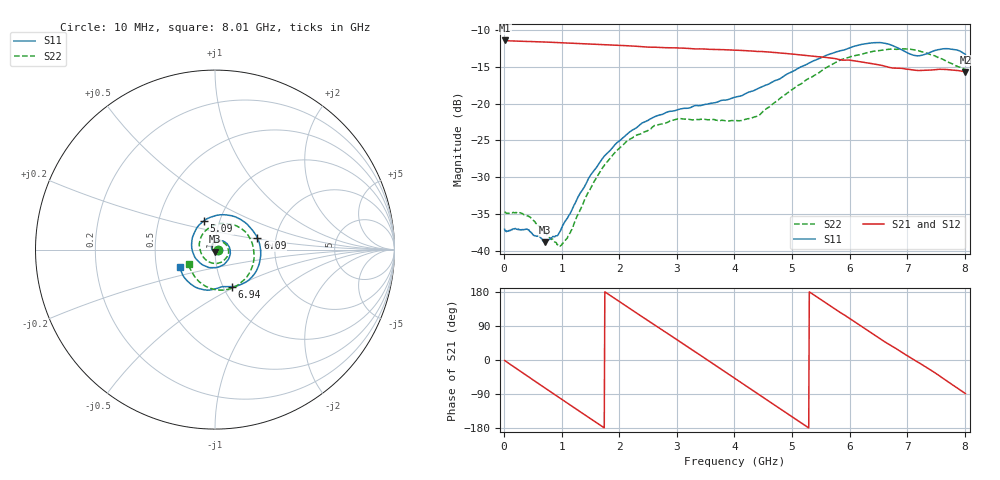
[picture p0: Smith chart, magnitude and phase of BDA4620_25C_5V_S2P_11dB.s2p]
!Agilent Technologies,E5071B,MY42404982,A.09.10
!Date: Wed May 06 09:00:28 2026
!Data & Calibration Information:
!Freq	S11:SOLT2(ON)	S21:SOLT2(ON)	S12:SOLT2(ON)	S22:SOLT2(ON)
# Hz S RI R 50
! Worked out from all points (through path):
!   801 points, 10 MHz to 8.01 GHz, reference 50 ohm
!   highest |S21| = -11.44 dB at 10 MHz (marker M1); lowest = -15.7 dB at 8.01 GHz (marker M2)
!   group delay of S21, straight-line fit = 280 ps
!   lowest |S11| = -38.9 dB at 710 MHz (marker M3), VSWR 1.02, Z = 49.9 - j1.14 ohm
!   |S11| at or under -10 dB: start of sweep to end of sweep
!   |S22| runs from -39.4 to -12.6 dB; largest |S21 - S12| = 0.0012
!   S11 on the Smith chart (normalised r, x): 10 MHz: 1.03, -0.00; 5.09 GHz: 0.84, +0.28; 6.09 GHz: 1.60, +0.22; 6.94 GHz: 1.10, -0.48; 8.01 GHz: 0.67, -0.13
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1e7  0.014 -0.00093  0.2679 -0.0057  0.2683 -0.00581  0.0184 -0.00107
4.2e8  0.00997 -0.00968  0.1902 -0.1827  0.1905 -0.1833  0.0137 -0.0103
7.1e8  -0.000638 -0.0114  0.073 -0.251  0.073 -0.2516  0.0034 -0.013
9.9e8  -0.0131 -0.00478  -0.056 -0.2525  -0.0564 -0.253  -0.0086 -0.00671
1.35e9  -0.0192 0.0169  -0.1938 -0.1659  -0.1939 -0.1661  -0.0153 0.0128
1.67e9  -0.0066 0.0397  -0.249 -0.035  -0.2494 -0.0351  -0.00637 0.034
1.94e9  0.0162 0.0507  -0.2346 0.0825  -0.2349 0.0828  0.0129 0.0455
2.33e9  0.0569 0.0407  -0.1257 0.2093  -0.126 0.2096  0.0475 0.0393
2.68e9  0.0831 0.00493  0.017 0.24  0.0173 0.2403  0.0703 0.0138
3.39e9  0.0393 -0.0885  0.2275 0.0585  0.2279 0.0583  0.046 -0.0628
4.01e9  -0.0738 -0.082  0.1521 -0.1728  0.1523 -0.1732  -0.0452 -0.0619
4.52e9  -0.1306 0.0203  -0.0419 -0.2209  -0.042 -0.2213  -0.0874 0.021
5.09e9  -0.0617 0.1606  -0.2006 -0.0772  -0.2012 -0.0771  -0.0185 0.1303
5.35e9  0.0163 0.1924  -0.2089 0.0192  -0.2091 0.0194  0.0468 0.1443
5.68e9  0.1305 0.1749  -0.1589 0.1271  -0.1588 0.1276  0.1337 0.1246
6.09e9  0.2367 0.0646  -0.0341 0.1918  -0.0343 0.1923  0.2099 0.0263
6.39e9  0.2505 -0.062  0.0641 0.1751  0.0641 0.1753  0.2157 -0.0652
6.68e9  0.1853 -0.1721  0.1322 0.1164  0.1326 0.1169  0.1793 -0.1495
6.94e9  0.0957 -0.2064  0.1648 0.0507  0.1653 0.0506  0.116 -0.2049
7.19e9  0.0375 -0.2074  0.1666 -0.0179  0.1671 -0.0181  0.0333 -0.2262
7.58e9  -0.077 -0.2205  0.1229 -0.1187  0.1234 -0.1189  -0.0799 -0.186
8.01e9  -0.1932 -0.0963  0.0042 -0.164  0.00436 -0.1645  -0.1474 -0.0826
